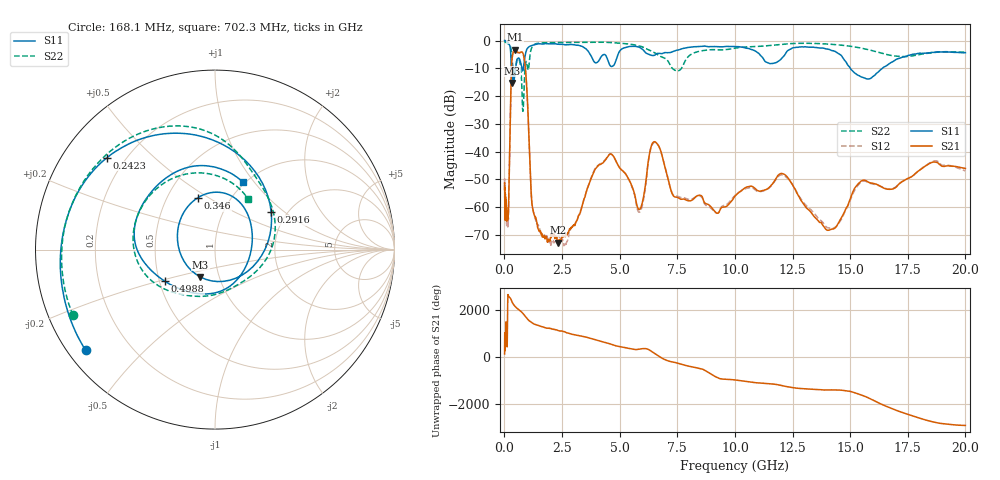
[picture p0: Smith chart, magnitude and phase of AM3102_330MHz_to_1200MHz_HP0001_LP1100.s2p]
! Date/Time: Tue, Sep 11, 2018 5:10 PM
! Network Analyzer: Agilent Technologies E8362B Rev: A.07.50.63
! Sweep from 0.010 to 20.000 GHz, 1601 Points, Sweep Type: LOG
! Power Supply: 4.950 V, 0.001 A
# Hz S DB R 50
!freq MagS11 AngS11 MagS21 AngS21 MagS12 AngS12 MagS22 AngS22
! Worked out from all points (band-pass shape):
!   1601 points, 10 MHz to 20 GHz, reference 50 ohm
!   highest |S21| = -3.31 dB at 455.8 MHz (marker M1); lowest = -72.8 dB at 2.314 GHz (marker M2)
!   |S21| within 3 dB of the highest: 335.1 MHz to 856.8 MHz (521.7 MHz wide, 87.5 % of centre)
!   lowest |S11| = -15.2 dB at 316.2 MHz (marker M3), VSWR 1.42, Z = 40.7 - j12.8 ohm
!   |S11| at or under -10 dB: 362.6 MHz to 494.1 MHz (131.4 MHz wide, 30.7 % of centre); 757 MHz to 822.7 MHz (65.7 MHz wide, 8.32 % of centre); 15.01 GHz to 16.4 GHz (1.392 GHz wide, 8.87 % of centre)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
!   |S22| runs from -25.5 to -0.3 dB; largest |S21 - S12| = 0.012
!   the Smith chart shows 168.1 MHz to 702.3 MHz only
!   S11 on the Smith chart (normalised r, x): 168.1 MHz: 0.05, -0.34; 242.3 MHz: 0.13, +0.36; 291.6 MHz: 1.66, +0.81; 346 MHz: 0.71, +0.45; 498.8 MHz: 0.53, -0.21; 702.3 MHz: 0.97, +0.88
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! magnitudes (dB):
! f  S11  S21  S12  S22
! 10 MHz  0.0  -51.2  -54.1  -0.3
! 35.55 MHz  0.0  -60.0  -60.0  -0.5
! 126.4 MHz  -0.4  -63.0  -63.2  -1.0
! 168.1 MHz  -0.8  -62.3  -65.6  -1.2
! 242.3 MHz  -2.0  -34.9  -35.0  -1.8
! 291.6 MHz  -8.5  -14.3  -14.3  -3.4
! 316.2 MHz  -15.2  -8.3  -8.3  -5.7
! 346 MHz  -10.3  -5.7  -5.7  -7.8
! 447.2 MHz  -12.8  -3.3  -3.4  -11.8
! 455.8 MHz  -12.4  -3.3  -3.3  -11.4
! 498.8 MHz  -9.6  -3.5  -3.6  -9.2
! 702.3 MHz  -7.8  -4.2  -4.3  -9.4
! 806 MHz  -10.7  -4.6  -4.7  -25.5
! 1.207 GHz  -1.8  -59.4  -59.4  -2.3
! 1.59 GHz  -1.3  -69.3  -69.7  -0.9
! 2.314 GHz  -1.3  -72.8  -69.9  -0.7
! 4.543 GHz  -8.3  -41.1  -41.0  -0.7
! 5.652 GHz  -2.1  -55.4  -55.7  -1.6
! 6.58 GHz  -4.9  -36.7  -36.8  -4.8
! 7.552 GHz  -3.4  -56.6  -56.2  -10.9
! 14.07 GHz  -3.2  -68.3  -67.4  -1.3
! 20 GHz  -4.4  -46.0  -47.0  -4.2
